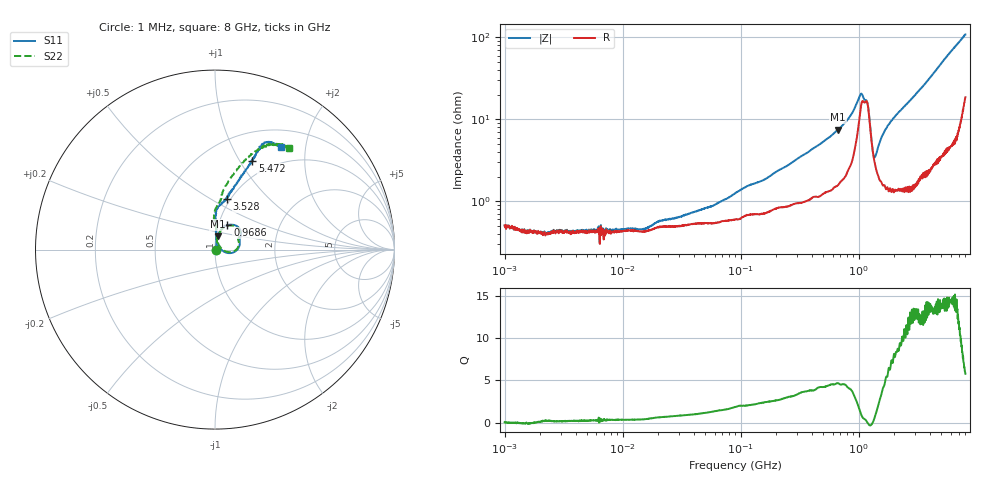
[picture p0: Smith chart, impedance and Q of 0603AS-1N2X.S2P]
!s-Parameter Generated by FASTRON Sdn. Bhd.
!FASTRON P/N : 0603AS-1N2X
!Keysight Technologies: E5071C_MY46733604_B.14.02
!Date: Tue Oct 24 10:17:14 2023
!Version  :Rev01  Tue Oct 24 10:17:14 2023
!Data & Calibration Information:
!Freq  S11:SOLT2(ON)  S21:SOLT2(ON)  S12:SOLT2(ON)  S22:SOLT2(ON)
!PortZ  Port1:50+j0  Port2:50+j0
!When reading reference impedance value at option line is always used.
! Remarks : This data is being provided solely for informational purposes.
# Hz S dB R 50
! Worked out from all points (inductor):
!   1601 points, 1 MHz to 8 GHz, reference 50 ohm
!   read as one part in series: L = 1.56 nH near 250.5 MHz
!   highest Q = 4.55 at 666.5 MHz (marker M1), where L = 1.74 nH
!   self-resonance near 1.184 GHz
!   S11 on the Smith chart (normalised r, x): 1 MHz: 1.01, -0.00; 968.6 MHz: 1.10, +0.31; 3.528 GHz: 0.96, +0.59; 5.472 GHz: 0.82, +1.14; 8 GHz: 0.74, +1.57
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1000000  -45.41 -4.0  -0.04 -0.1  -0.04 -0.0  -45.28 -0.1
1577378  -48.38 -16.1  -0.04 -0.0  -0.04 0.0  -46.16 -27.9
2311589  -48.07 9.4  -0.04 -0.1  -0.05 -0.0  -51.69 18.7
2922607  -48.34 9.9  -0.04 -0.1  -0.05 -0.0  -48.60 1.2
4479405  -47.62 11.1  -0.04 -0.1  -0.04 -0.0  -49.21 15.0
8407329  -47.22 14.3  -0.04 -0.1  -0.04 -0.1  -47.78 15.6
1.526847e7  -53.55 -15.2  -0.03 -0.1  -0.05 -0.2  -44.86 17.3
2.00676e7  -45.93 29.0  -0.04 -0.2  -0.05 -0.1  -44.99 38.7
5.928355e7  -41.83 55.1  -0.05 -0.4  -0.06 -0.4  -41.81 52.2
8.994653e7  -38.31 63.1  -0.05 -0.7  -0.06 -0.6  -38.84 60.2
1.598705e8  -35.61 71.2  -0.07 -1.0  -0.08 -1.0  -35.13 67.1
4.006501e8  -27.11 77.1  -0.12 -2.2  -0.13 -2.2  -27.13 76.4
6.665231e8  -22.32 78.5  -0.20 -3.9  -0.21 -3.9  -22.37 77.5
9.68578e8  -16.30 63.3  -0.68 -7.5  -0.69 -7.5  -16.43 61.9
1.047189e9  -14.90 40.8  -1.34 -6.6  -1.35 -6.6  -15.21 39.7
1.14826e9  -16.85 15.5  -1.42 -1.8  -1.42 -1.8  -17.09 19.6
1.341815e9  -31.34 43.7  -0.36 -0.0  -0.37 -0.1  -29.93 35.7
1.52743e9  -24.34 84.0  -0.27 -2.4  -0.27 -2.5  -24.41 79.6
1.7949e9  -20.60 87.3  -0.28 -4.3  -0.28 -4.4  -20.83 85.7
3.527775e9  -10.74 77.0  -0.84 -11.2  -0.84 -11.3  -11.06 83.2
5.472309e9  -5.42 67.1  -2.31 -20.5  -2.30 -20.6  -5.32 70.5
8e9  -3.36 57.3  -5.42 -28.7  -5.41 -29.2  -3.14 54.0
